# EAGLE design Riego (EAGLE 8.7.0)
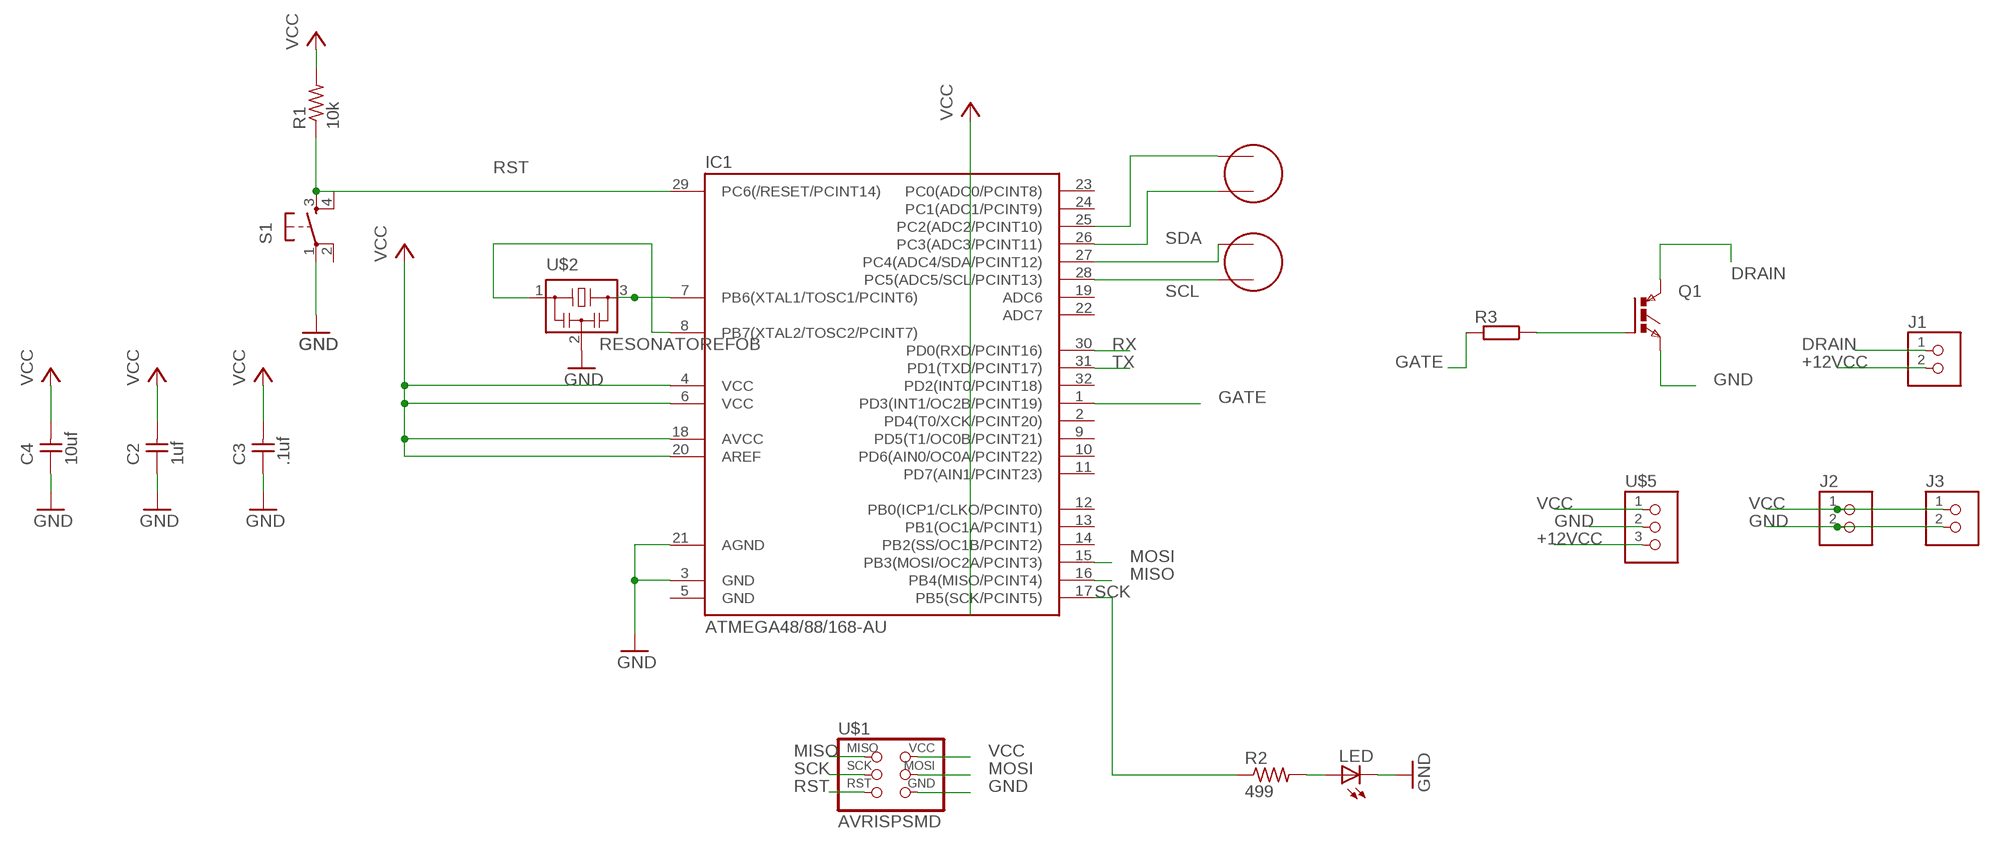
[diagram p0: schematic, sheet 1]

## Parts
C2  1uf  UNPOLARIZED_CAPACITOR1206  [1206]
C3  .1uf  UNPOLARIZED_CAPACITOR1206  [1206]
C4  10uf  UNPOLARIZED_CAPACITOR1206  [1206]
IC1  ATMEGA48/88/168-AU  [TQFP32-08]
J1  TERM-1X02-ADAFRUIT  [3.5MMTERM]
J2  TERM-1X02-ADAFRUIT  [3.5MMTERM]
J3  TERM-1X02-ADAFRUIT  [3.5MMTERM]
LED  LED1206  [1206]
Q1  IGBTTO252  [TO252]
R1  10k  RESISTOR1206  [1206]
R2  499  RESISTOR1206  [1206]
R3  SMR  [SMR]
S1  6MM_SWITCH6MM_SWITCH  [6MM_SWITCH]
U$1  AVRISPSMD  [2X03SMD]
U$2  RESONATOREFOB  [EFOBM]
U$3  ELECTRET  [ELECTRET_2742PBJ-A]
U$5  TERM-1X03'-FABLAB'  [ED555DS-3DS]
U$6  ELECTRET  [ELECTRET_2742PBJ-A]

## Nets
+12VCC: J1.2 U$5.3
DRAIN: J1.1 Q1.2(C)
GATE: IC1.1(PD3(INT1/OC2B/PCINT19)) R3.2
GND: C2.1 C3.1 C4.1 IC1.3(GND) IC1.21(AGND) J2.2 J3.2 LED.2(C) Q1.3(E) S1.1(P) U$1.6(GND) U$2.2 U$5.2
MISO: IC1.16(PB4(MISO/PCINT4)) U$1.1(MISO)
MOSI: IC1.15(PB3(MOSI/OC2A/PCINT3)) U$1.4(MOSI)
N$1: IC1.8(PB7(XTAL2/TOSC2/PCINT7)) U$2.1
N$4: Q1.1(G) R3.1
N$6: IC1.26(PC3(ADC3/PCINT11)) U$6.P$2
N$7: IC1.25(PC2(ADC2/PCINT10)) U$6.P$1
N$9: IC1.7(PB6(XTAL1/TOSC1/PCINT6)) U$2.3
N$23: LED.1(A) R2.2
RST: IC1.29(PC6(/RESET/PCINT14)) R1.1 S1.3(S) U$1.5(RST)
RX: IC1.30(PD0(RXD/PCINT16))
SCK: IC1.17(PB5(SCK/PCINT5)) R2.1 U$1.3(SCK)
SCL: IC1.28(PC5(ADC5/SCL/PCINT13)) U$3.P$2
SDA: IC1.27(PC4(ADC4/SDA/PCINT12)) U$3.P$1
TX: IC1.31(PD1(TXD/PCINT17))
VCC: C2.2 C3.2 C4.2 IC1.4(VCC) IC1.6(VCC) IC1.18(AVCC) IC1.20(AREF) J2.1 J3.1 R1.2 U$1.2(VCC) U$5.1
Unconnected: IC1.2(PD4(T0/XCK/PCINT20)) IC1.9(PD5(T1/OC0B/PCINT21)) IC1.10(PD6(AIN0/OC0A/PCINT22)) IC1.11(PD7(AIN1/PCINT23)) IC1.12(PB0(ICP1/CLKO/PCINT0)) IC1.13(PB1(OC1A/PCINT1)) IC1.14(PB2(SS/OC1B/PCINT2)) IC1.19(ADC6) IC1.22(ADC7) IC1.23(PC0(ADC0/PCINT8)) IC1.24(PC1(ADC1/PCINT9)) IC1.32(PD2(INT0/PCINT18)) S1.2(P1) S1.4(S1)

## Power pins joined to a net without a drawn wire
GND: IC1.5(GND)

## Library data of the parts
C2-C4 = ng:UNPOLARIZED_CAPACITOR: unpolarized_capacitor
IC1 = atmega8:ATMEGA48/88/168
J1-J3 = fab:TERM-1X02: 3.5mm terminal block, 2 positions ED555-2DS as found in the fablab inventory.
LED = ng:LED
Q1 = IGBT:IGBT: IGBT
R1 R2 = ng:RESISTOR
R3 = resistor-shunt:SMR: SMD SHUNT RESISTOR; OC_FARNELL: unknown; OC_NEWARK: unknown
S1 = ng:6MM_SWITCH: OMRON SWITCH
U$1 = fab:AVRISP
U$2 = fab:RESONATOR
U$3 U$6 = fab:ELECTRET
U$5 = fab:TERM-1X03: 3.5mm terminal block, 3 positions ED555-3DS as found in the fablab inventory. Made by Zaerc.

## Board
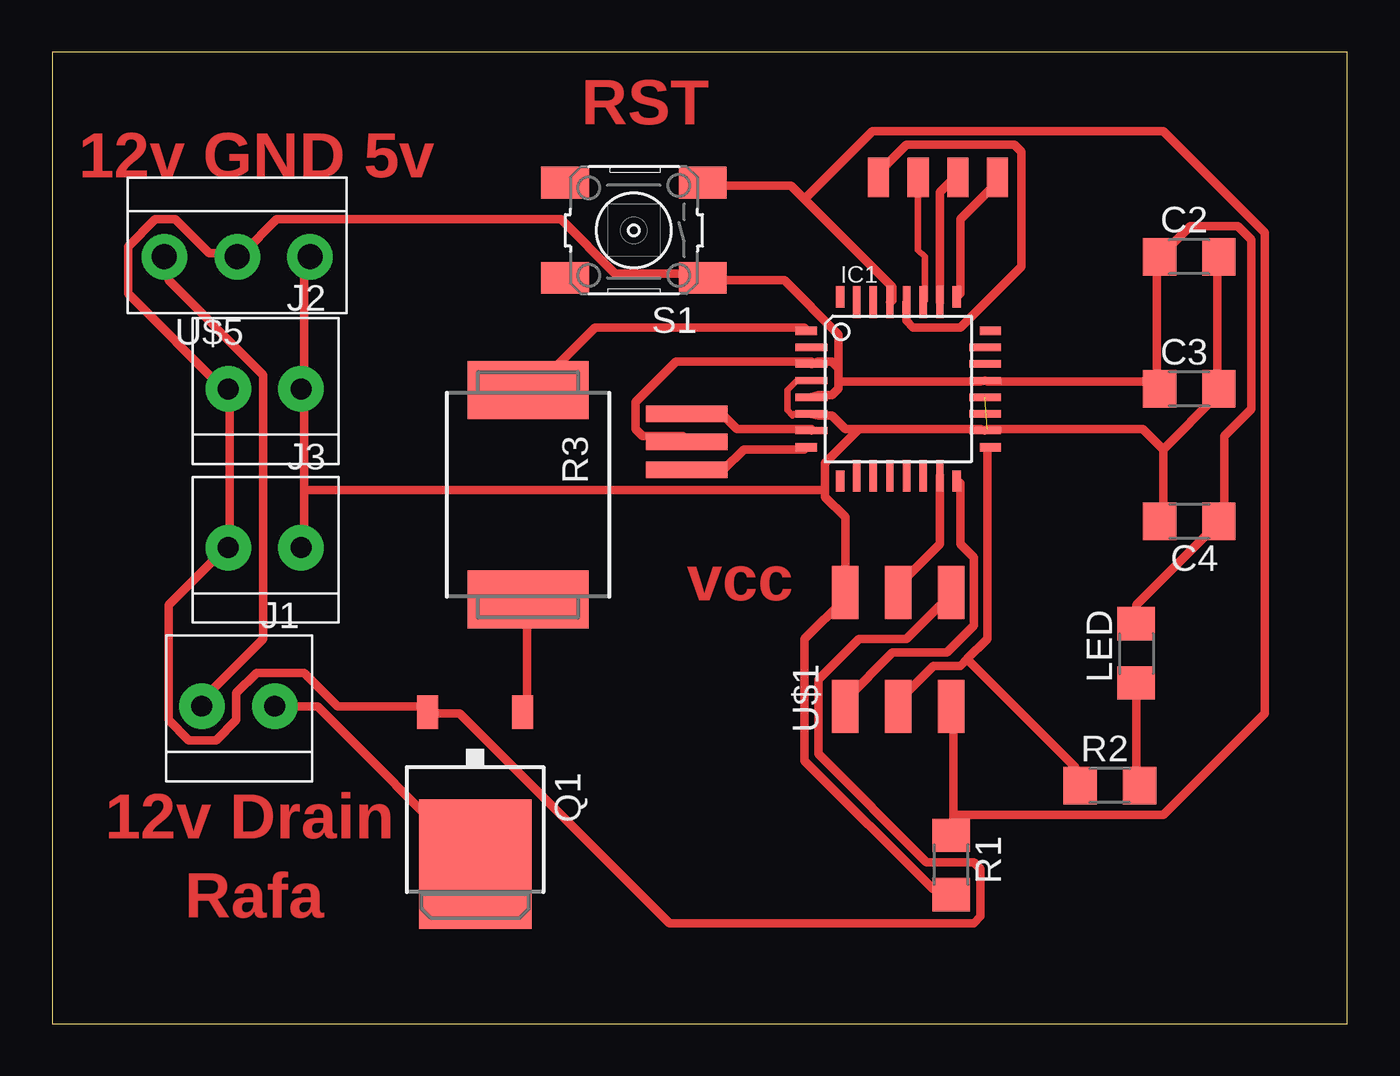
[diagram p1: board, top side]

Size 62.21 x 46.66 mm. Coordinates in mm from the lower left corner, seen from the top.
Outline: 0,0 62.21,0 62.21,46.66 0,46.66 0,0
Copper layers (1*16): Top 0.035mm / dielectric 1.5mm / Bottom 0.035mm
Design rules "default *": minimum track width 0.4mm, minimum drill 0.4mm, track to track 0.25mm, track to pad 0.25mm, pad to pad 0.25mm, via to via 0.25mm, smd to smd 0.25mm, copper to edge 40mil, drill to drill 6mil, minimum pad ring 10mil, minimum via ring 8mil, stop-mask expansion 4mil, vias tented up to drill 0mil, thermal gap 10mil

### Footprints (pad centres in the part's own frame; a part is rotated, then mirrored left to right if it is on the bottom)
1206 = smd 1.6 x 1.803: 1 -1.422,0; 2 1.422,0
TQFP32-08 = smd 1.016 x 0.406: 1 -4.42,2.8; 8 -4.42,-2.8; 17 4.42,-2.8; 24 4.42,2.8 | smd 1.524 x 0.356: 2 -4.166,2; 3 -4.166,1.2; 4 -4.166,0.4; 5 -4.166,-0.4; 6 -4.166,-1.2; 7 -4.166,-2; 18 4.166,-2; 19 4.166,-1.2; 20 4.166,-0.4; 21 4.166,0.4; 22 4.166,1.2; 23 4.166,2 | smd 0.406 x 1.016: 9 -2.8,-4.42; 16 2.8,-4.42; 25 2.8,4.42; 32 -2.8,4.42 | smd 0.356 x 1.524: 10 -2,-4.166; 11 -1.2,-4.166; 12 -0.4,-4.166; 13 0.4,-4.166; 14 1.2,-4.166; 15 2,-4.166; 26 2,4.166; 27 1.2,4.166; 28 0.4,4.166; 29 -0.4,4.166; 30 -1.2,4.166; 31 -2,4.166
3.5MMTERM = drill 1 pad 2.184: 1 1.8,0; 2 -1.7,0
TO252 = smd 1 x 1.6: 1 -2.28,-4.8; 3 2.28,-4.8 | smd 5.4 x 6.2: 2 0,2.5
SMR = smd 2.8 x 5.8: 1 5.029,0; 2 -5.029,0
6MM_SWITCH = smd 2.286 x 1.524: 1 -3.302,2.286; 2 3.302,2.286; 3 -3.302,-2.286; 4 3.302,-2.286
2X03SMD = smd 2.54 x 1.27: 1 -2.54,2.54; 2 2.92,2.54; 3 -2.54,0; 4 2.92,0; 5 -2.54,-2.54; 6 2.92,-2.54
EFOBM = smd 0.8 x 3.9: 1 -1.35,0; 2 0,0; 3 1.35,0
ELECTRET_2742PBJ-A = smd 1.016 x 1.905: P$1 -0.953,0; P$2 0.953,0
ED555DS-3DS = drill 1.2 pad 2.184: 1 -3.5,0; 2 0,0; 3 3.5,0

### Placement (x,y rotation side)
C2  54.61,36.83 0 top
C3  54.61,30.48 0 top
C4  54.61,24.13 180 top
IC1  40.64,30.48 0 top
J1  8.89,15.24 0 top
J2  10.16,30.48 0 top
J3  10.16,22.86 0 top
LED  52.07,17.78 90 top
Q1  20.32,10.16 180 top
R1  43.18,7.62 270 top
R2  50.8,11.43 0 top
R3  22.86,25.4 270 top
S1  27.94,38.1 180 top
U$1  40.64,17.78 90 top
U$2  30.48,27.94 90 top
U$3  40.64,40.64 180 top
U$5  8.89,36.83 180 top
U$6  44.45,40.64 180 top

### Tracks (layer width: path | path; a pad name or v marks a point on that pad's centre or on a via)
+12VCC
  Top 0.4: U$5.3 5.59,36.67 5.59,35.7 10.14,31.15 10.14,18.48 7.22,15.55 J1.2
DRAIN
  Top 0.4: J1.1 10.79,15.22 12.74,15.22 20.22,7.75 Q1.2
GATE
  Top 0.4: IC1.1 36.15,33.42 26.07,33.42 23.14,30.5 R3.2
GND
  Top 0.4: LED.2 52.07,20.1 55.97,24 C4.1 56.3,24.32 56.3,28.23 57.59,29.52 57.59,37.65 56.95,38.3 54.67,38.3 53.37,37 C2.1 53.05,36.67 53.05,30.82 | 53.05,30.82 53.05,30.5 C3.1 53.05,30.82 | 37.77,31.48 37.77,30.82 | 37.77,30.82 37.77,30.5 37.45,30.18 36.8,30.18 IC1.5 | 37.77,31.48 37.45,31.8 36.8,31.8 IC1.3 36.47,31.8 29.97,31.8 28.02,29.85 28.02,28.55 28.34,28.23 30.3,28.23 U$2.2 | 37.77,30.82 44.59,30.82 IC1.21 44.92,30.82 53.05,30.82 | 37.77,31.48 37.77,33.1 35.17,35.7 31.27,35.7 S1.1 30.95,36.02 27.05,36.02 24.45,38.62 10.79,38.62 9.17,37 U$5.2 8.85,37 7.54,37 5.92,38.62 4.95,38.62 3.65,37.33 3.65,35.05 8.2,30.5 J2.2 8.52,30.18 8.52,23.02 J3.2 8.2,22.7 5.59,20.1 5.59,14.57 6.57,13.6 7.87,13.6 8.85,14.57 8.85,15.88 9.82,16.85 12.1,16.85 13.72,15.22 17.95,15.22 Q1.3 18.27,14.9 19.57,14.9 29.64,4.83 44.27,4.83 44.59,5.15 44.59,7.42 44.27,7.75 41.99,7.75 36.8,12.95 36.8,16.52 38.74,18.48 41.02,18.48 42.97,20.43 U$1.6
MISO
  Top 0.4: IC1.16 43.62,25.95 43.62,23.02 44.27,22.38 44.27,19.12 42.97,17.82 40.37,17.82 38.09,15.55 U$1.1
MOSI
  Top 0.4: IC1.15 42.65,26.27 42.65,23.02 40.37,20.75 U$1.4
N$1
  Top 0.4: IC1.8 36.15,27.57 33.22,27.57 32.24,26.6 30.62,26.6 U$2.1
N$4
  Top 0.4: Q1.1 22.82,15.22 22.82,20.1 R3.1
N$6
  Top 0.4: IC1.26 42.65,34.73 42.65,39.92 43.3,40.58 U$6.P$2
N$7
  Top 0.4: IC1.25 43.62,35.05 43.62,38.62 45.57,40.58 U$6.P$1
N$9
  Top 0.4: IC1.7 36.47,28.55 32.9,28.55 32.24,29.2 30.62,29.2 U$2.3
N$23
  Top 0.4: LED.1 52.07,11.65 R2.2
RST
  Top 0.4: 43.3,10.03 43.3,15.22 U$1.5 | 43.3,10.03 43.3,9.05 R1.1 | 36.15,39.6 35.49,40.25 31.27,40.25 S1.3 | 36.15,39.6 40.37,35.38 40.37,34.73 IC1.29 | 43.3,10.03 53.37,10.03 58.24,14.9 58.24,37.98 53.37,42.85 39.4,42.85 36.15,39.6
SCK
  Top 0.4: 43.95,17.5 43.62,17.18 42.32,17.18 40.7,15.55 U$1.3 | 43.95,17.5 44.92,18.48 44.92,27.57 IC1.17 | 43.95,17.5 49.15,12.3 49.15,11.65 R2.1
SCL
  Top 0.4: IC1.28 41.02,34.4 41.02,33.75 41.34,33.42 43.62,33.42 46.55,36.35 46.55,41.88 46.22,42.2 41.02,42.2 39.72,40.9 U$3.P$2
SDA
  Top 0.305: U$3.P$1 41.59,37.15 41.91,36.83 41.91,34.72 IC1.27
VCC  (1 unrouted)
  Top 0.305: IC1.4 35.77,30.88 35.31,30.42 35.31,29.46 35.56,29.21 35.63,29.28 IC1.6
  Top 0.4: 12.1,25.62 12.1,30.18 J2.1 12.1,30.5 12.1,36.67 U$5.1 | 12.1,25.62 12.1,23.02 J3.1 | R1.2 42.97,6.45 42.32,6.45 36.15,12.62 36.15,18.48 38.09,20.43 U$1.2 38.09,20.75 38.09,24.32 37.12,25.3 37.12,25.62 | 38.74,28.55 38.09,28.55 37.45,29.2 36.8,29.2 IC1.6 | 38.74,28.55 44.59,28.55 IC1.18 44.92,28.55 52.4,28.55 53.37,27.57 | 53.37,27.57 53.37,24.32 C4.2 | 53.37,27.57 55.97,30.18 C3.2 55.97,30.5 55.97,36.67 C2.2 | 37.12,25.62 37.12,26.93 38.74,28.55 | 37.12,25.62 12.1,25.62

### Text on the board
Top: RST | 12v GND 5v | vcc | 12v Drain | Rafa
